FUNCTION_BLOCK FB_RPMSource
VAR_INPUT
	t : LREAL;
END_VAR
VAR_OUTPUT
	rpm : LREAL;
END_VAR
VAR
	m_maxrpm: UDINT;
	m_minrpm: UDINT;
	m_operationcycle: LREAL;
	m_cyclepos: LREAL;
END_VAR

m_cyclepos := ABS(SIN(t/m_operationcycle * PI));

rpm := m_cyclepos * (m_maxrpm-m_minrpm) + m_minrpm;

METHOD FB_init : BOOL
VAR_INPUT
	bInitRetains : BOOL; // if TRUE, the retain variables are initialized (warm start / cold start)
	bInCopyCode : BOOL;  // if TRUE, the instance afterwards gets moved into the copy code (online change)
	maxrpm  : UDINT;
	minrpm: UDINT;
	operationcycle : LREAL;
END_VAR
m_maxrpm := maxrpm;
m_minrpm := minrpm;
m_operationcycle := operationcycle;
END_METHOD

END_FUNCTION_BLOCK
